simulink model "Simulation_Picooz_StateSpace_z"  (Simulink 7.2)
settings: Solver=ode1  StartTime=0.0  StopTime=60  FixedStep=0.002  RelTol=1e-3
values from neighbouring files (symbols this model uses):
  Az = [0.8544 0.9806]    [Synthese_controleurPicooz_StateSpace_Integrateur.m]
  Bz = [-0.0207 0.0659]'    [Synthese_controleurPicooz_StateSpace_Integrateur.m]
  Cz = [-0.0319   -0.0107]    [Synthese_controleurPicooz_StateSpace_Integrateur.m]
undefined symbols (not defined in the file or in its folder): DiscIntNeverNeededParam
libraries: simulink x1, cstblocks x1

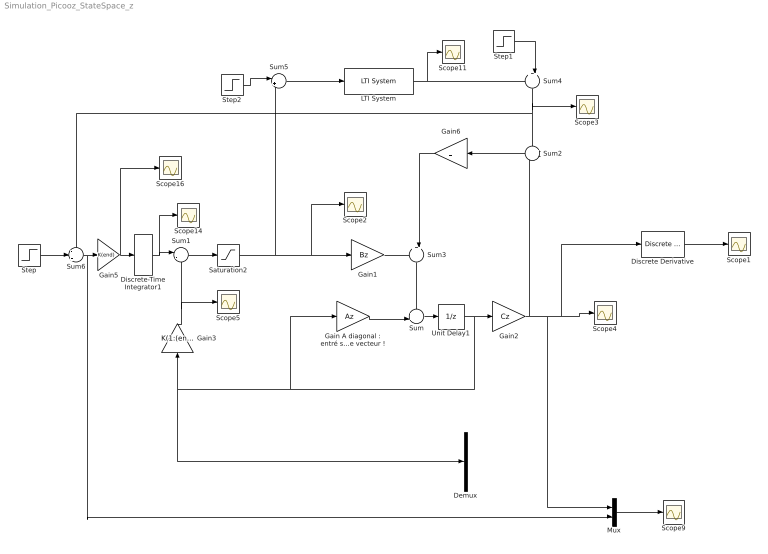
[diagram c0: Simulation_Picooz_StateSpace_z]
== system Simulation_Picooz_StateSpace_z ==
  Demux : Demux  Outputs=2
  Discrete Derivative : simulink/Discrete/Discrete Derivative  SystemSampleTime=-1  gainval=1.0  ICPrevScaledInput=0.0  OutMin=[]  OutMax=[]  OutDataType=sfix(16)  OutScaling=2^-10  DoSatur=off
  Discrete-Time Integrator1 : DiscreteIntegrator  gainval=1  SampleTime=.002  OutDataType=fixdt(1,32,20)  SaturateOnIntegerOverflow=on  LimitOutput=on  UpperSaturationLimit=200000  LowerSaturationLimit=-200000  ICPrevOutput=DiscIntNeverNeededParam  ICPrevScaledInput=DiscIntNeverNeededParam
  "Gain A diagonal : entré sous forme de vecteur !" : Gain  Gain=Az  ParameterDataType=sfix(16)  ParameterScaling=2^0  OutDataType=sfix(16)  OutScaling=2^0
  Gain1 : Gain  Gain=Bz  Multiplication=Matrix(K*u)  ParameterDataType=sfix(16)  ParameterScaling=2^0  OutDataType=sfix(16)  OutScaling=2^0
  Gain2 : Gain  Gain=Cz  Multiplication=Matrix(K*u)  ParameterDataType=sfix(16)  ParameterScaling=2^0  OutDataType=sfix(16)  OutScaling=2^0
  Gain3 : Gain  Orientation=up  Gain=K(1:(end-1))  Multiplication=Matrix(K*u)  ParameterDataType=sfix(16)  ParameterScaling=2^0  OutDataType=sfix(16)  OutScaling=2^0
  Gain5 : Gain  Gain=K(end)  Multiplication=Matrix(K*u)  ParameterDataType=sfix(16)  ParameterScaling=2^0  OutDataType=sfix(16)  OutScaling=2^0
  Gain6 : Gain  Orientation=left  Gain=L'  Multiplication=Matrix(K*u)  ParameterDataType=sfix(16)  ParameterScaling=2^0  OutDataType=sfix(16)  OutScaling=2^0
  LTI System : cstblocks/LTI System  SystemSampleTime=-1  sys=Picooz_Mrotor_z  IC=[]
  Mux : Mux  Inputs=2
  Saturation2 : Saturate  UpperLimit=11999  LowerLimit=0  OutDataType=sfix(16)  OutScaling=2^0
  Scope{1..5,9,11,14,16} (9 alike) : Scope
  Step : Step  Time=0  After=100  SampleTime=.002
  Step1 : Step  Time=0  After=1000  SampleTime=.002
  Step2 : Step  Time=0  After=6000  SampleTime=.002
  Sum : Sum  Inputs=++|  OutDataType=sfix(16)  OutScaling=2^0
  Sum1 : Sum  Inputs=|--  OutDataType=sfix(16)  OutScaling=2^0
  Sum2 : Sum  Orientation=left  Inputs=+-  OutDataType=sfix(16)  OutScaling=2^0
  Sum3 : Sum  Orientation=down  Inputs=++|  OutDataType=sfix(16)  OutScaling=2^0
  Sum4 : Sum  Orientation=down  Inputs=++|  OutDataType=sfix(16)  OutScaling=2^0
  Sum5 : Sum  Inputs=|++  OutDataType=sfix(16)  OutScaling=2^0
  Sum6 : Sum  Inputs=-++  OutDataType=sfix(16)  OutScaling=2^0
  Unit Delay1 : UnitDelay  X0=[0 0]  SampleTime=-1
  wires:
  Sum/1 -> Unit Delay1/1
  "Gain A diagonal : entré sous forme de vecteur !"/1 -> Sum/2
  Gain2/1 -> Discrete Derivative/1, Scope4/1, Mux/1, Sum2/2
  Sum1/1 -> Saturation2/1
  Gain1/1 -> Sum3/1
  Sum6/1 -> Mux/2, Gain5/1
  Unit Delay1/1 -> Gain2/1, Gain3/1, Demux/1, "Gain A diagonal : entré sous forme de vecteur !"/1
  LTI System/1 -> Scope11/1, Sum4/1
  Discrete Derivative/1 -> Scope1/1
  Mux/1 -> Scope9/1
  Sum4/1 -> Sum2/1, Sum6/1, Scope3/1
  Sum3/1 -> Sum/1
  Gain3/1 -> Sum1/2, Scope5/1
  Gain5/1 -> Discrete-Time Integrator1/1, Scope16/1
  Discrete-Time Integrator1/1 -> Sum1/1, Scope14/1
  Sum2/1 -> Gain6/1
  Gain6/1 -> Sum3/2
  Step/1 -> Sum6/2
  Sum5/1 -> LTI System/1
  Step1/1 -> Sum4/2
  Saturation2/1 -> Gain1/1, Scope2/1, Sum5/2
  Step2/1 -> Sum5/1
